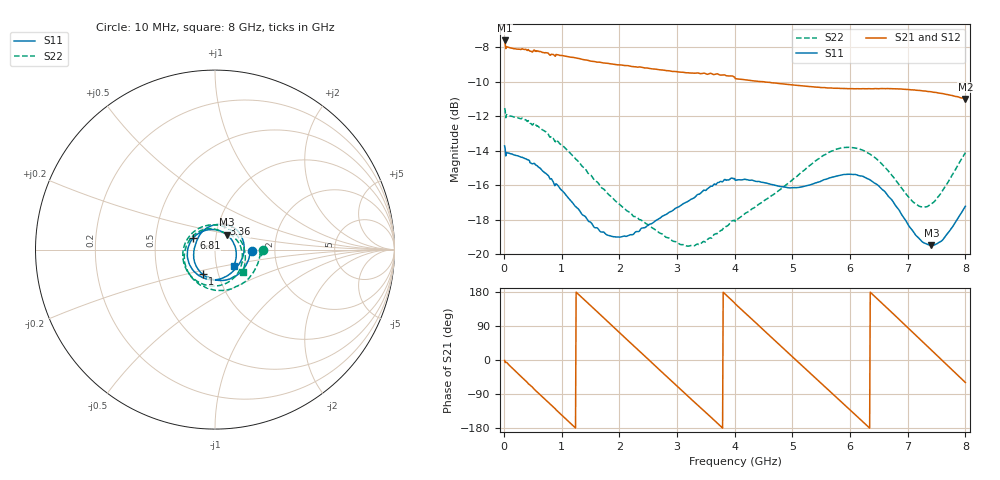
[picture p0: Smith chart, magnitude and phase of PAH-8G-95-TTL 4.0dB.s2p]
! MTS Systemtechnik GmbH
! S-Parameters
! Model: PAH-8G/95-TTL
! Attenuation Step: 4.0dB
! Rohde & Schwarz ZVB8 2Ports - Version 4.11 - 1145.1010k08 SN: 100119
! S2P File Measurements:
! S11 S21 S12 S22
# HZ  S  DB  R  50.00
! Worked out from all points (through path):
!   800 points, 10 MHz to 8 GHz, reference 50 ohm
!   highest |S21| = -7.62 dB at 10 MHz (marker M1); lowest = -11.0 dB at 8 GHz (marker M2)
!   group delay of S21, straight-line fit = 394 ps
!   lowest |S11| = -19.5 dB at 7.41 GHz (marker M3), VSWR 1.24, Z = 56.2 + j9.5 ohm
!   |S11| at or under -10 dB: start of sweep to end of sweep
!   |S22| runs from -19.5 to -11.5 dB; largest |S21 - S12| = 0.0052
!   S11 on the Smith chart (normalised r, x): 10 MHz: 1.52, -0.02; 1 GHz: 0.84, -0.24; 3.36 GHz: 1.06, +0.30; 6.81 GHz: 0.78, +0.11; 8 GHz: 1.21, -0.22
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1e7  -13.72 -1.5  -7.62 -1.2  -7.52 -1.1  -11.53 -1.1
5.5e8  -14.82 -66.5  -8.23 -80.9  -8.23 -80.8  -12.52 -69.1
1e9  -16.29 -117.0  -8.49 -145.4  -8.48 -145.3  -13.66 -122.2
1.35e9  -17.67 -151.7  -8.71 164.8  -8.71 164.8  -14.88 -160.4
1.67e9  -18.68 -177.7  -8.88 119.5  -8.89 119.8  -16.06 168.5
1.95e9  -19.00 162.5  -9.02 79.2  -9.03 79.3  -16.96 144.1
2.35e9  -18.63 137.1  -9.15 23.4  -9.15 23.5  -17.99 115.3
2.68e9  -17.95 115.3  -9.31 -23.8  -9.31 -23.5  -18.72 94.2
3.03e9  -17.25 91.8  -9.44 -73.4  -9.45 -73.7  -19.38 76.0
3.36e9  -16.53 70.8  -9.50 -119.2  -9.52 -119.6  -19.40 62.8
3.7e9  -15.86 48.9  -9.55 -166.9  -9.58 -166.8  -18.79 49.9
4.01e9  -15.71 26.1  -9.83 148.0  -9.83 148.0  -18.10 34.2
4.56e9  -15.89 -11.0  -10.03 70.6  -10.05 70.6  -16.79 4.3
4.96e9  -16.15 -35.9  -10.18 14.2  -10.19 14.1  -15.80 -20.0
5.34e9  -15.94 -59.4  -10.30 -38.9  -10.32 -38.9  -14.77 -46.5
5.88e9  -15.38 -102.1  -10.40 -114.7  -10.42 -114.7  -13.82 -93.5
6.29e9  -15.60 -143.9  -10.41 -172.6  -10.44 -172.6  -14.09 -137.2
6.67e9  -16.66 170.1  -10.41 133.2  -10.41 133.3  -15.20 175.0
6.81e9  -17.26 151.1  -10.42 113.1  -10.42 113.1  -15.79 155.1
7.09e9  -18.65 108.2  -10.48 72.5  -10.48 72.6  -16.96 109.3
7.41e9  -19.48 51.9  -10.59 26.1  -10.59 26.1  -17.08 51.0
8e9  -17.22 -40.2  -11.00 -59.4  -11.00 -59.3  -14.11 -38.8
